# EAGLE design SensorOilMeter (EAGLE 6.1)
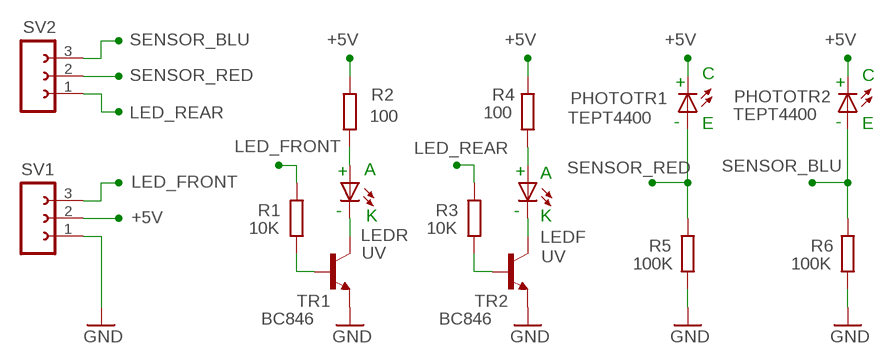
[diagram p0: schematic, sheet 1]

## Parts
LEDF  UV  LED5MM_F  [LED5MM]
LEDR  UV  LED5MM_F  [LED5MM]
PHOTOTR1  TEPT4400  LED3MM_F  [LED3MM]
PHOTOTR2  TEPT4400  LED3MM_F  [LED3MM]
R1  10K  R-EU_R1206_L  [R1206_L]
R2  100  R-EU_R1206  [R1206]
R3  10K  R-EU_R1206  [R1206]
R4  100  R-EU_R1206_L  [R1206_L]
R5  100K  R-EU_R0805  [R0805]
R6  100K  R-EU_R0805  [R0805]
SV1  FE03-1"  [FE03-1]
SV2  FE03-1"  [FE03-1]
TR1  BC846  -NPN-BC846  [SOT23_L]
TR2  BC846  -NPN-BC846  [SOT23_L]

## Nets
+5V: PHOTOTR1.K(C) PHOTOTR2.K(C) R2.1 R4.1 SV1.2
GND: R5.1 R6.1 SV1.1 TR1.2(E) TR2.2(E)
LED_FRONT: R1.2 SV1.3
LED_REAR: R3.2 SV2.1
N$1: LEDR.K(C) TR1.3(C)
N$2: LEDR.A R2.2
N$3: LEDF.A R4.2
N$4: LEDF.K(C) TR2.3(C)
N$5: R1.1 TR1.1(B)
N$6: R3.1 TR2.1(B)
SENSOR_BLU: PHOTOTR2.A R6.2 SV2.3
SENSOR_RED: PHOTOTR1.A R5.2 SV2.2

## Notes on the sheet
- C | C
- + | +
- - | E | - | E
- + | A | + | A
- - | -
- K | K

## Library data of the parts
LEDF LEDR PHOTOTR1 PHOTOTR2 = 00-LIVIO:LED: LEDS
R1-R6 = 00-LIVIO:R-EU_: RESISTOR, European symbol
SV1 SV2 = 02-con-lsta-F:FE03-1: FEMALE HEADER
TR1 TR2 = 00-LIVIO:*-NPN-: NPN Transistror

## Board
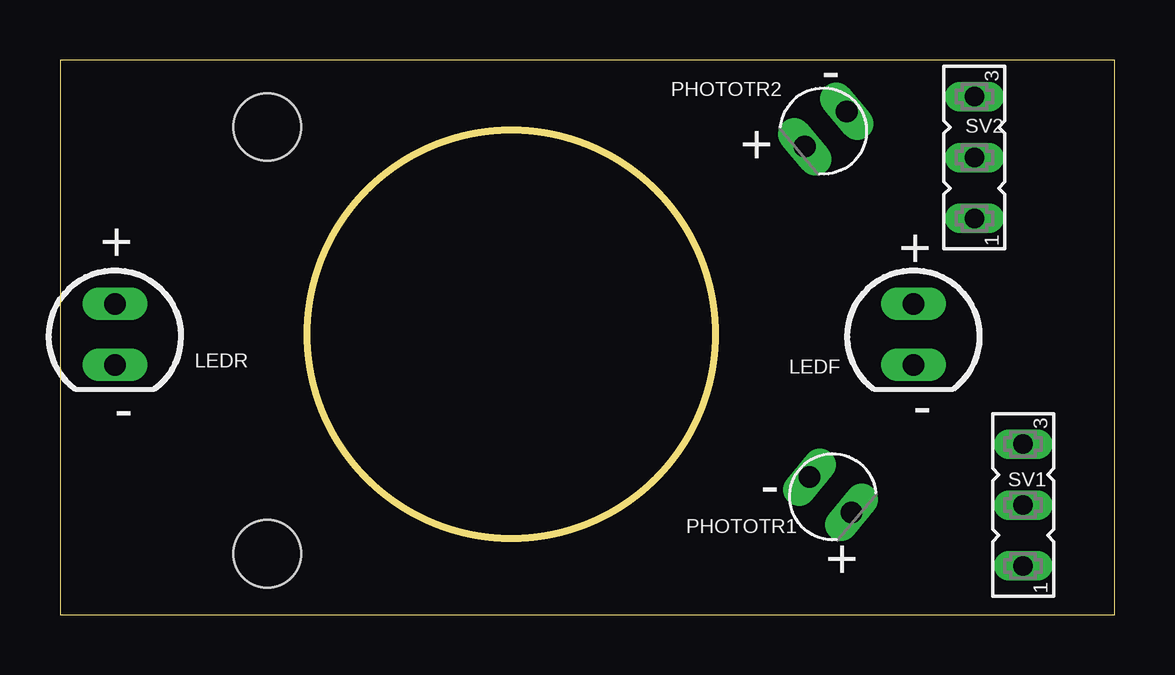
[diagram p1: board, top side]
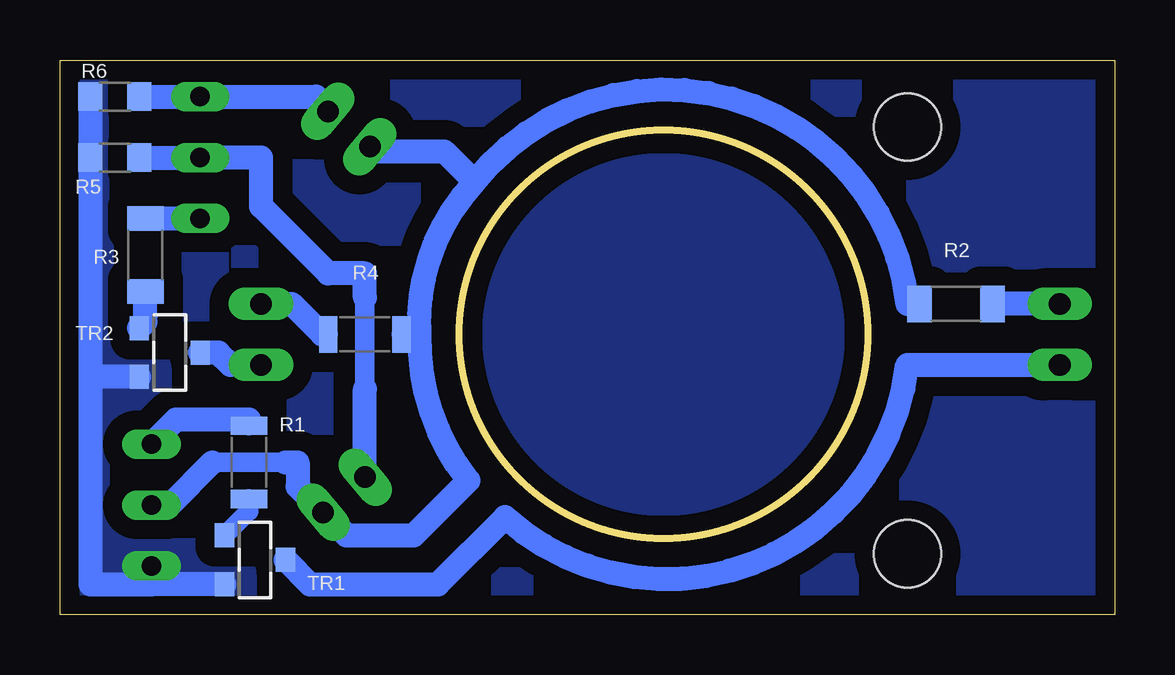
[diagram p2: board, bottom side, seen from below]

Size 43.94 x 23.11 mm. Coordinates in mm from the lower left corner, seen from the top.
Outline: 0,0 43.94,0 43.94,23.11 0,23.11 0,0
Outline: circle at 18.8,11.68 radius 8.5
Copper layers (1*16): Top 0.035mm / dielectric 1.5mm / Bottom 0.035mm
Design rules: minimum track width 10mil, minimum drill 0.6mm, track to track 8mil, track to pad 8mil, pad to pad 8mil, via to via 8mil, smd to smd 8mil, copper to edge 31mil, drill to drill 8mil, minimum pad ring 5mil, minimum via ring 8mil, stop-mask expansion 4mil, vias tented up to drill 0mil, thermal gap 41mil
Holes 2.8 mm at 8.64,20.32 8.64,2.54

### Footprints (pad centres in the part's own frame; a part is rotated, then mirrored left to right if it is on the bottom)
LED5MM = drill 0.9 long: A -1.27,0; K 1.27,0
LED3MM = drill 0.9 long: A -1.016,0; K 1.27,0
R1206_L = smd 0.762 x 1.524: 1 -1.524,0; 2 1.524,0
R1206 = smd 1.016 x 1.524: 1 -1.524,0; 2 1.524,0
R0805 = smd 1 x 1.2: 1 -1.016,0; 2 1.016,0
FE03-1 = drill 0.813 long: 1 -2.54,0; 2 0,0; 3 2.54,0
SOT23_L = smd 1 x 0.8: 1 -1.016,-1.27; 2 1.016,-1.27; 3 0,1.27

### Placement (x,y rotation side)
LEDF  35.56,11.68 270 top
LEDR  2.29,11.68 270 top
PHOTOTR1  32,5.08 320 top
PHOTOTR2  32,20.32 220 top
R1  36.07,6.35 90 bottom
R2  6.6,12.95 0 bottom
R3  40.39,14.99 90 bottom
R4  31.24,11.68 180 bottom
R5  41.66,19.05 0 bottom
R6  41.66,21.59 0 bottom
SV1  40.13,4.57 90 top
SV2  38.1,19.05 90 top
TR1  35.81,2.29 270 bottom
TR2  39.37,10.92 270 bottom

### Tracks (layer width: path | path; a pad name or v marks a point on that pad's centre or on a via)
+5V
  Bottom 0.813: 37.59,6.35 37.34,6.35 34.8,6.35 34.54,6.35 | R4.1 29.46,11.68
  Bottom 1: 26.67,18.03 27.94,19.3 30.99,19.3 31.03,19.35 PHOTOTR2.K | 26.67,18.03 arc135 8.64,12.95 R2.1 | 37.59,6.35 39.37,4.57 SV1.2 | 28.96,11.68 arc-40 26.92,5.59 29.21,3.3 32,3.3 33.02,4.32 | 28.96,11.68 arc46 26.67,18.03 | 34.54,6.35 34.04,6.35 34.04,5.33 33.02,4.32 | 33.02,4.32 33.02,4.26 | 33.02,4.26 PHOTOTR1.K 33.02,4.26 | 33.02,4.26 33.02,4.32 | 29.46,11.68 28.96,11.68
GND
  Bottom 1: SV1.1 40.13,1.78 | SV1.1 40.13,1.78 | TR1.2 40.13,1.27 | 40.13,1.27 40.13,1.52 40.13,1.78 | 42.67,9.91 R5.1 R6.1 | 42.67,9.91 42.67,1.27 40.13,1.27 | 40.13,1.27 40.13,1.78 | TR2.2 42.67,9.91 | SV1.1 40.13,1.78
  pour Bottom (isolate 0.8, rank 6, no thermals): -1,-1 44.94,-1 44.94,24.11 -1,24.11
LED_FRONT
  Bottom 0.813: R1.2 36.07,8.13
  Bottom 1: 36.07,8.13 39.12,8.13 SV1.3
LED_REAR
  Bottom 1: R3.2 SV2.1
N$1
  Bottom 1: TR1.3 33.53,1.27 28.19,1.27 25.4,4.06 arc-125 8.64,10.41 LEDR.K
N$2
  Bottom 1: LEDR.A 2.16,12.95 R2.2
N$3
  Bottom 0.813: 33.02,11.68 R4.2
  Bottom 1: LEDF.A 34.29,12.95 33.02,11.68
N$4
  Bottom 1: LEDF.K 36.83,10.41 37.34,10.92 TR2.3
N$5
  Bottom 0.813: R1.1 36.07,4.32 TR1.1
N$6
  Bottom 1: TR2.1 40.39,12.19 40.39,12.45 R3.1
SENSOR_BLU
  Bottom 1: R6.2 SV2.3 37.59,21.59 33.27,21.59 32.87,21.18 32.78,21.1 PHOTOTR2.A
SENSOR_RED
  Bottom 0.813: 31.24,9.4 31.24,13.21
  Bottom 1: R5.2 SV2.2 35.56,19.05 35.56,17.02 32.77,14.22 31.24,14.22 31.24,13.21 | 31.24,9.4 31.24,6.1 31.23,6.08 PHOTOTR1.A

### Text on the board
tNames: - | + | + | + | - | - | - | +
